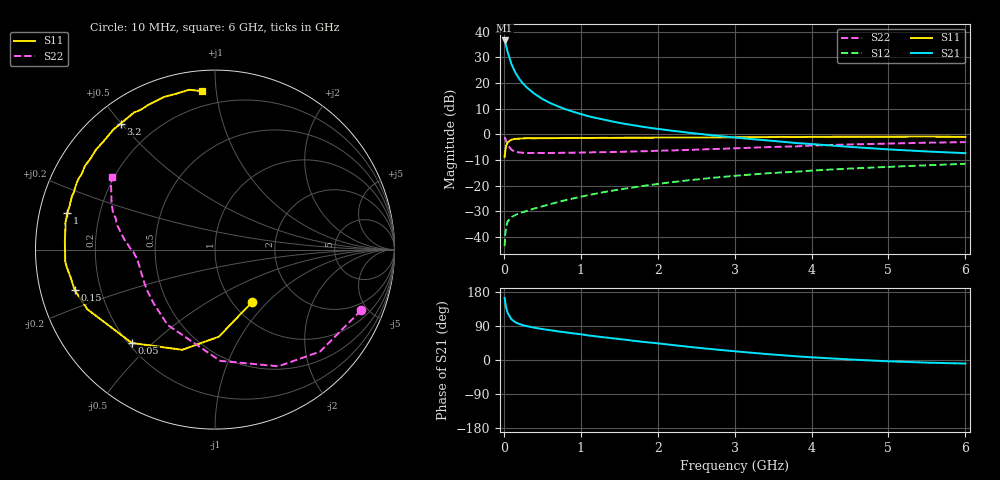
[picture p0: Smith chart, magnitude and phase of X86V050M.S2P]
! SIEMENS Small Signal Semiconductors
! BFP136W
! Si NPN RF Bipolar Junction Transistor in SOT343
! VCE = 6 V  IC = 50 mA
! Common Emitter S-Parameters:  September  1994
# GHz  S  MA  R  50
!  f  S11  S21  S12  S22
! GHz  MAG  ANG  MAG  ANG  MAG  ANG  MAG  ANG
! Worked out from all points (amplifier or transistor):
!   40 points, 10 MHz to 6 GHz, reference 50 ohm
!   highest |S21| = 36.5 dB at 10 MHz (marker M1)
!   |S21| within 3 dB of that: start of sweep to 37.78 MHz
!   unconditionally stable (mu >= 1): 743 MHz to 2.917 GHz
!   at 200 MHz: K = 0.53, MSG = 26.2 dB, |S12| = -30.8 dB
!   at 1.5 GHz: K = 1.11, MAG = 11.0 dB, |S12| = -21.5 dB
!   at 6 GHz: K = 0.96, MSG = 2.1 dB, |S12| = -11.5 dB
!   S11 on the Smith chart (normalised r, x): 10 MHz: 1.22, -0.82; 50 MHz: 0.21, -0.43; 150 MHz: 0.10, -0.14; 1 GHz: 0.08, +0.12; 3.2 GHz: 0.08, +0.50; 6 GHz: 0.11, +0.91
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0.01  0.3576 -54.6  67.17 163.8  0.0066 73.1  0.8814 -22.6
0.02  0.4854 -87.4  60.16 149.6  0.0118 63.0  0.8159 -44.1
0.03  0.5874 -108.1  53.1 138.6  0.0157 53.6  0.7398 -61.5
0.05  0.6968 -131.7  40 123.7  0.0201 41.5  0.6207 -87.3
0.1  0.7847 -154.9  23.08 107.1  0.0244 33.6  0.4958 -122.1
0.15  0.814 -164.0  15.88 99.6  0.0267 33.0  0.4553 -138.5
0.2  0.8194 -169.2  11.99 95.0  0.0289 34.0  0.442 -147.9
0.25  0.8309 -172.9  9.687 91.8  0.0305 36.0  0.4363 -153.9
0.3  0.8372 -175.5  8.113 89.3  0.0321 37.7  0.4318 -158.0
0.4  0.8356 180.0  6.124 85.1  0.036 40.6  0.4308 -163.4
0.5  0.8378 176.7  4.883 81.6  0.0393 43.7  0.431 -166.9
0.6  0.839 174.4  4.072 78.8  0.0435 46.2  0.4319 -169.1
0.7  0.8421 171.8  3.513 75.6  0.0474 48.6  0.434 -170.7
0.8  0.8471 169.8  3.076 73.1  0.052 50.3  0.4355 -172.1
1  0.8475 166.0  2.479 68.0  0.0606 52.7  0.4397 -174.2
1.1  0.8458 163.2  2.246 64.7  0.0652 53.4  0.4428 -175.1
1.5  0.8517 156.4  1.668 55.3  0.0837 54.9  0.4537 -178.0
2.2  0.8595 143.9  1.164 39.4  0.1171 52.7  0.4841 177.0
3.2  0.8767 126.8  0.81 19.5  0.1633 45.3  0.5444 168.1
4.5  0.8967 108.6  0.567 1.4  0.2145 34.4  0.6331 155.6
5.5  0.9021 99.2  0.462 -6.9  0.2486 26.4  0.6839 147.9
6  0.8863 94.8  0.428 -9.4  0.2656 22.1  0.7028 144.6
